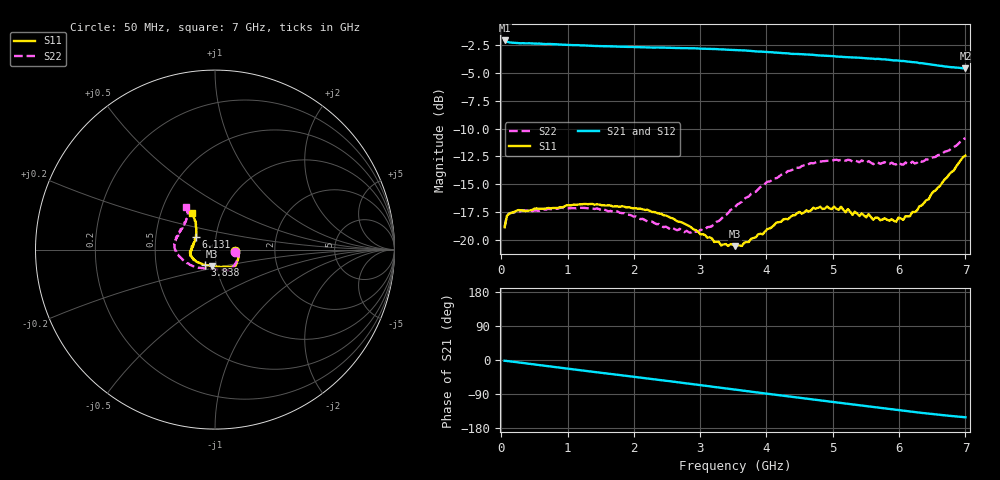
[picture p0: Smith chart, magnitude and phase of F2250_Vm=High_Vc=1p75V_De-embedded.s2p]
! Integrated Device Technology
! Corporate Headquarters
! 6024 Silver Creek Valley Road
! San Jose, CA 95138  USA
! Phone:  1-408-284-8200
! Toll Free:  1-800-223-1366
! Webpage:  http://www.idt.com/
! Timing and RF Division
! 515 Groton Road, Suite 102
! Westford, MA 01886-6024
! Device:  F2250
! Description: Voltage Variable RF Attenuator
! Frequency:  50.0 -  6000.00 MHz
! Package:  3x3 mm Thin QFN Plastic Package: 16 pin
! Ports:  2 RF, 3 DC
!  Pin  1  = GND
!  Pin  2  = NC
!  Pin  3  = RF1  = Port 1
!  Pin  4  = NC
!  Pin  5  = GND
!  Pin  6  = GND
!  Pin  7  = GND
!  Pin  8  = GND
!  Pin  9  = NC
!  Pin 10  = RF2  = Port 2
!  Pin 11  = NC
!  Pin 12  = GND
!  Pin 13  = GND
!  Pin 14  = VCNTRL
!  Pin 15  = VDD
!  Pin 16  = VMODE
! Vcntrl:  1.750 Volts
! Vmode:  +3.300 Volts
! Vdd:  +3.30  Volts
! Current:  1.327 mA
! Data:  The device was measured on a the F2250 evaluation board which has
!  individual transmission lines to the RF pins.  Data was collected
!  using a calibrated network analyzer.  The evaluation board was
!  de-embedded using a TRL calibration technique.
!  The reference plane is the edge of the package pin.
! Misc:  SN 10
!  Action Tracker AT0258
! Date Measured:  2014-11-26
! Date:  2015-10-15  MJV
! Note:
!  Integrated Device Technology supplies this data as a sample of measured
!  data at the package pin for this product.  Your particular data for this
!  product may vary.
!  Data was taken at 25 degrees C.
!  Integrated Device Technology reserves the right to change this data at anytime.
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# GHz S dB R 50
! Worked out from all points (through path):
!   201 points, 50 MHz to 7 GHz, reference 50 ohm
!   highest |S21| = -2.10 dB at 50 MHz (marker M1); lowest = -4.6 dB at 7 GHz (marker M2)
!   group delay of S21, straight-line fit = 60.7 ps
!   lowest |S11| = -20.5 dB at 3.525 GHz (marker M3), VSWR 1.21, Z = 47.4 - j8.82 ohm
!   |S11| at or under -10 dB: start of sweep to end of sweep
!   |S22| runs from -19.3 to -10.9 dB; largest |S21 - S12| = 0.0024
!   S11 on the Smith chart (normalised r, x): 50 MHz: 1.26, -0.02; 3.838 GHz: 0.88, -0.15; 6.131 GHz: 0.80, +0.12; 7 GHz: 0.72, +0.31
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0.05  -18.85 -4.5  -2.10 -1.9  -2.10 -1.9  -18.83 -5.9
0.08475  -17.83 -4.4  -2.21 -2.6  -2.21 -2.6  -17.80 -5.5
0.2585  -17.31 -9.9  -2.34 -6.4  -2.34 -6.4  -17.45 -12.6
1.2315  -16.78 -36.6  -2.54 -27.8  -2.54 -27.8  -17.12 -48.3
1.75275  -16.98 -43.2  -2.65 -38.9  -2.65 -39.0  -17.43 -59.8
2.37825  -17.62 -46.9  -2.73 -52.4  -2.74 -52.4  -18.56 -72.9
2.969  -19.24 -61.5  -2.82 -65.5  -2.83 -65.5  -19.25 -100.6
3.3165  -20.48 -84.7  -2.89 -73.4  -2.88 -73.4  -18.10 -123.9
3.525  -20.55 -101.0  -2.96 -78.1  -2.96 -78.1  -17.05 -135.6
3.83775  -19.76 -124.6  -3.08 -85.1  -3.07 -85.1  -15.67 -150.6
4.32425  -18.13 -149.8  -3.26 -95.9  -3.26 -95.9  -13.81 -169.3
4.7065  -17.10 -163.6  -3.39 -104.3  -3.41 -104.3  -13.12 -179.3
5.1235  -17.01 -174.3  -3.56 -113.4  -3.57 -113.4  -12.81 170.5
5.29725  -17.75 -179.5  -3.62 -117.1  -3.60 -117.2  -12.95 167.0
5.332  -17.46 178.9  -3.63 -117.9  -3.63 -118.0  -12.86 166.0
5.50575  -17.96 173.8  -3.70 -121.7  -3.71 -121.7  -13.05 161.9
5.5405  -17.67 171.7  -3.72 -122.4  -3.73 -122.5  -12.93 160.4
5.61  -18.19 171.5  -3.74 -123.9  -3.75 -123.9  -13.19 159.4
5.85325  -18.26 159.9  -3.84 -129.1  -3.85 -129.2  -13.17 152.1
6.13125  -17.88 146.2  -4.00 -135.1  -3.99 -135.2  -13.17 144.4
6.54825  -15.55 130.1  -4.31 -143.7  -4.30 -143.8  -12.55 130.9
7  -12.43 122.6  -4.61 -151.1  -4.61 -151.2  -10.85 124.4
